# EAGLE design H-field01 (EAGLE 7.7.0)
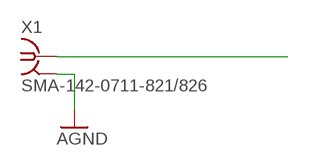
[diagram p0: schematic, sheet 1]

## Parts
X1  SMA-142-0711-821/826  [J502-ND-142-0711-821/826]

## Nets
AGND: X1.G@1 X1.G@2 X1.G@3 X1.G@4
N$1: X1.1

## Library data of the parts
X1 = con-coax:SMA-: SMA 50 Ohm End Launch Jack Receptacle - Round Contact; MF: JOHNSON COMPONENTS; MPN: 142-0711-821; OC_FARNELL: 1019328; OC_NEWARK: 16F3627

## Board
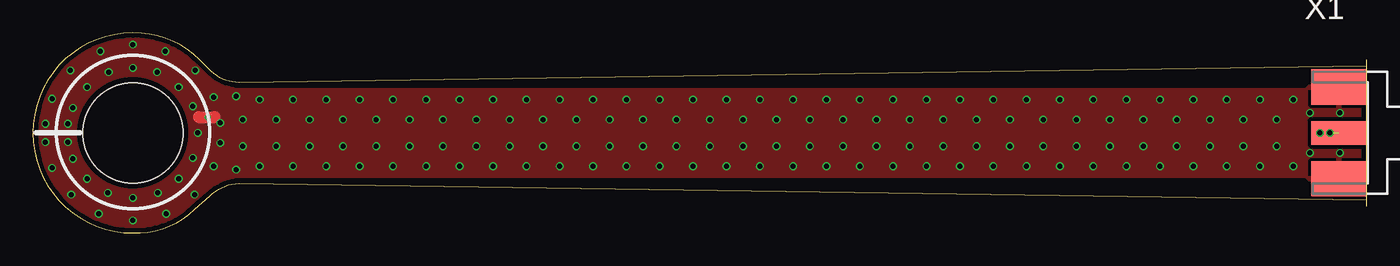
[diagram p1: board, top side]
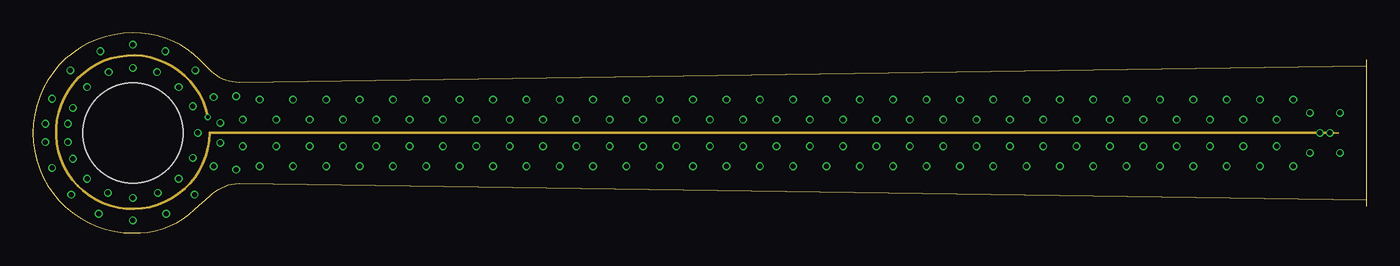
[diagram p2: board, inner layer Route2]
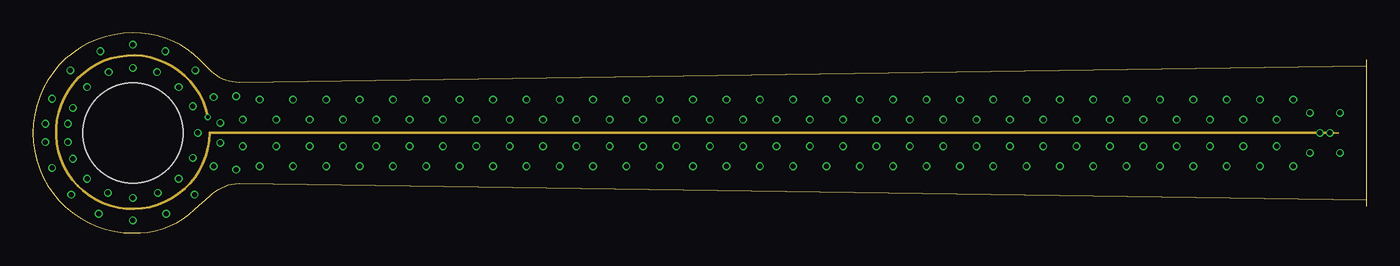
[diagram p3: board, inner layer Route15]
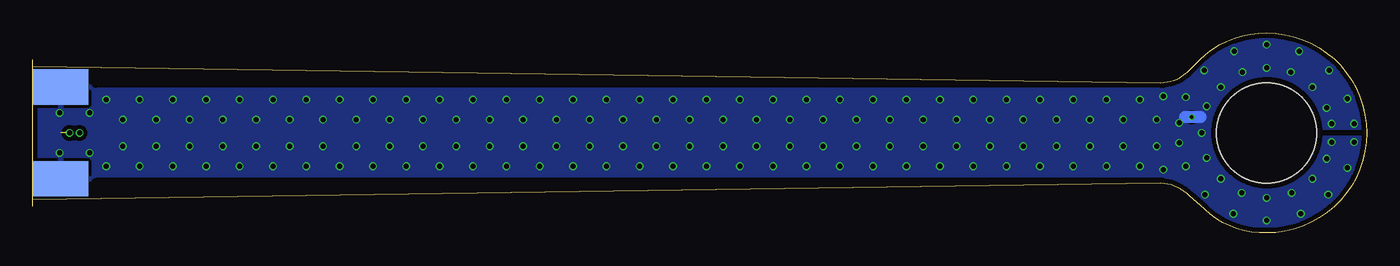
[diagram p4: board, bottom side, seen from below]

Size 101.6 x 15.24 mm. Coordinates in mm from the lower left corner, seen from the top.
Outline: 0,7.62 arc90 7.62,0 arc45 12.34,1.8 13.5,2.83 arc-42 15.7,3.79 101.6,2.54 101.6,12.7 15.7,11.45 arc-42 13.63,12.29 12.72,13.19 arc45 7.62,15.24 arc90 0,7.62
Copper layers (1+2*15+16): Top 0.0356mm / dielectric 0.1702mm / Route2 0.0178mm / dielectric 47mil / Route15 0.0178mm / dielectric 0.1702mm / Bottom 0.0356mm
Design rules "default *": minimum track width 5mil, minimum drill 10mil, track to track 12mil, track to pad 12mil, pad to pad 12mil, via to via 8mil, smd to smd 8mil, copper to edge 15mil, drill to drill 8mil, minimum pad ring 10mil, minimum via ring 4mil, stop-mask expansion 4mil, vias tented up to drill 0mil, thermal gap 10mil
Holes 7.62 mm at 7.62,7.62
tRestrict: area 3.6,3.6 to 11.6,11.6; 3 lines
bRestrict: area 3.6,3.6 to 11.6,11.6; 3 lines

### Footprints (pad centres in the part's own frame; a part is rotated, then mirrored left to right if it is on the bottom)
J502-ND-142-0711-821/826 = smd 4.191 x 1.778: 1 2.115,0 | smd 4.191 x 2.667: G@1 2.115,3.495; G@2 2.115,-3.495 | smd 4.191 x 2.667 bottom: G@3 2.115,3.495; G@4 2.115,-3.495

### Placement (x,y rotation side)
X1  101.6,7.62 180 top

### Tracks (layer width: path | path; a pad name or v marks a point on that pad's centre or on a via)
AGND  (via drill 0.38)
  Top 0.914: 12.64,8.83 13.84,8.83
  Bottom 0.914: 12.64,8.83 13.84,8.83
  other vias: 12.57,7.62 14.29,8.38 14.29,6.86 2.67,6.92 0.95,6.92 2.67,8.32 0.95,8.32 7.62,12.57 7.62,2.67 7.62,14.35 7.62,0.95 4.13,11.11 11.11,11.11 4.13,4.13 11.11,4.13 2.92,2.92 12.32,2.92 2.86,12.38 12.38,12.38 3.05,9.53 1.46,10.22 5.78,12.26 5.14,13.84 1.46,4.95 3.05,5.65 5.71,3.05 5.02,1.46 9.53,3.05 10.16,1.46 12.19,5.71 13.78,5.08 9.46,12.26 10.1,13.84 12.19,9.65 13.78,10.35 17.27,10.16 19.81,10.16 65.53,10.16 22.35,10.16 24.89,10.16 27.43,10.16 29.97,10.16 32.51,10.16 35.05,10.16 37.59,10.16 16,8.64 18.54,8.64 21.08,8.64 23.62,8.64 26.16,8.64 28.7,8.64 31.24,8.64 33.78,8.64 36.32,8.64 38.86,8.64 16,6.6 17.27,5.08 18.54,6.6 19.81,5.08 21.08,6.6 22.35,5.08 23.62,6.6 24.89,5.08 26.16,6.6 27.43,5.08 28.7,6.6 29.97,5.08 31.24,6.6 32.51,5.08 33.78,6.6 35.05,5.08 36.32,6.6 37.59,5.08 38.86,6.6 40.13,10.16 41.4,8.64 41.4,6.6 40.13,5.08 42.67,10.16 43.94,8.64 43.94,6.6 42.67,5.08 45.21,10.16 46.48,8.64 46.48,6.6 45.21,5.08 47.75,10.16 49.02,8.64 49.02,6.6 47.75,5.08 50.29,10.16 51.56,8.64 51.56,6.6 50.29,5.08 52.83,10.16 52.83,5.08 54.1,6.6 54.1,8.64 55.37,10.16 56.64,8.64 57.91,10.16 59.18,8.64 56.64,6.6 59.18,6.6 55.37,5.08 57.91,5.08 60.45,5.08 60.45,10.16 61.72,8.64 61.72,6.6 62.99,5.08 62.99,10.16 64.26,8.64 64.26,6.6 65.53,5.08 66.8,8.64 66.8,6.6 68.07,10.16 68.07,5.08 69.34,8.64 69.34,6.6 70.61,10.16 71.88,8.64 71.88,6.6 70.61,5.08 73.15,10.16 74.42,8.64 74.42,6.6 73.15,5.08 75.69,10.16 76.96,8.64 76.96,6.6 75.69,5.08 78.23,10.16 79.5,8.64 79.5,6.6 78.23,5.08 80.77,10.16 82.04,8.64 82.04,6.6 80.77,5.08 83.31,10.16 84.58,8.64 84.58,6.6 83.31,5.08 85.85,10.16 87.12,8.64 87.12,6.6 85.85,5.08 88.39,10.16 89.66,8.64 89.66,6.6 88.39,5.08 90.93,10.16 93.47,10.16 96.01,10.16 92.2,8.64 94.74,8.64 94.74,6.6 92.2,6.6 90.93,5.08 93.47,5.08 96.01,5.08 97.28,6.1 97.28,9.14 99.57,9.14 99.57,6.1 15.49,10.41 15.49,4.83
  pour Top: 0,0 104.14,0 104.14,15.24 0,15.24
  pour Bottom: 0,0 104.14,0 104.14,15.24 0,15.24
N$1  (via drill 0.38)  (1 unrouted)
  Route2 0.191: 99.06,7.62 v98.81,7.62 v98.04,7.62 13.46,7.62 arc-347 13.34,8.89
  Route15 0.191: 99.06,7.62 v98.81,7.62 v98.04,7.62 13.46,7.62 arc-347 13.34,8.89
N$3  (via drill 0.25)
  other vias: 13.34,8.83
